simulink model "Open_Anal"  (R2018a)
settings: Solver=ode113  StartTime=0.0  StopTime=25000  FixedStep=0.1  RelTol=1e-3  EnableMultiTasking=on
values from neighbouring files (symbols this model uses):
  atto = [0, 0, -0]'*d2r    [run.m]
  ini = [wb0; atto; Hco]    [run.m]
  Kq1 = I22*ww^2 - 3*wo2*(I11-I33)    [run.m]
  Kq2 = 2*I22*zet*ww    [run.m]
  Kqi = 0.0005    [run.m]
  Kr1 = (0.1*I11*I33*zet^2/Hy0) - sqrt( ((0.01^zet^4*I11^2*I33^2)/Hy0^2)+(4*I11*I33*zet^2) )    [run.m]
  Kr2 = 0.05*Kr1    [run.m]
  Kr3 = 0.04*zet*(Kr2-Hy0) * sqrt(abs(Hy0/(I11*I33)))    [run.m]
  Tbs = (wo2)*[-2*I32, 3*I31, -I12]'    [run.m]
  Ts = 0.001    [run.m]    (also in runf.m = 0.0005)
  wb0 = [0.0, -wo, 0.0]'    [run.m]
undefined symbols (not defined in the file or in its folder): Avf, Bvf, Cvf, den, DiscIntNeverNeededParam, Dvf, num, Spacecraft, Wheel_Dynamics
libraries: simulink x3

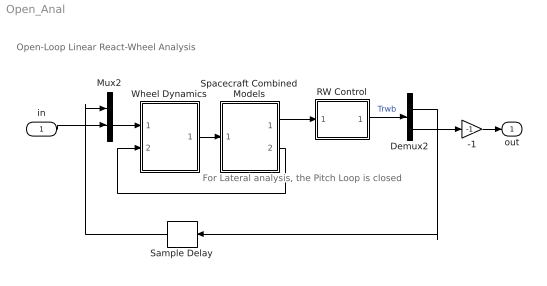
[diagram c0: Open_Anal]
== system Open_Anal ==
  note: Open-Loop Linear React-Wheel Analysis
  note: For Lateral analysis, the Pitch Loop is closed
  in : Inport
  -1 : Gain  Gain=-1
  Demux2 : Demux  Outputs=2
  Mux2 : Mux  Inputs=2
  RW Control : Subsystem
  Sample Delay : Delay  DelayLength=1  InputProcessing=Inherited  SampleTime=Ts
  Spacecraft Combined Models : Subsystem
  Wheel Dynamics : Subsystem
  out : Outport
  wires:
  -1/1 -> out/1
  Spacecraft Combined Models/2(wb) -> Wheel Dynamics/2(wb)
  Mux2/1 -> Wheel Dynamics/1(Twi)
  RW Control/1(Tc) -> Demux2/1  "Trwb"
  Spacecraft Combined Models/1(attit) -> RW Control/1(atti)
  Wheel Dynamics/1(Tcb) -> Spacecraft Combined Models/1(Trw)
  in/1 -> Mux2/2
  Demux2/2 -> -1/1
  Demux2/1 -> Sample Delay/1
  Sample Delay/1 -> Mux2/1

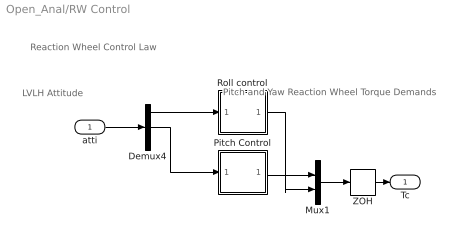
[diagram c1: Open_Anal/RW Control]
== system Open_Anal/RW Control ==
  note: Pitch and Yaw Reaction Wheel Torque Demands
  note: LVLH Attitude
  note: Reaction Wheel Control Law
  atti : Inport
  Demux4 : Demux  Outputs=3
  Mux1 : Mux  Inputs=2
  Pitch Control : Subsystem
  Roll control : Subsystem
  ZOH : ZeroOrderHold  SampleTime=Ts
  Tc : Outport
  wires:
  Demux4/1 -> Roll control/1(phi)
  Pitch Control/1(Tcy) -> Mux1/1
  Demux4/2 -> Pitch Control/1(the)
  Mux1/1 -> ZOH/1
  Roll control/1(Tcz) -> Mux1/2
  atti/1 -> Demux4/1
  ZOH/1 -> Tc/1

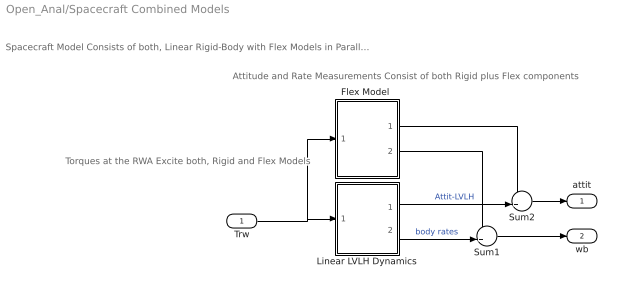
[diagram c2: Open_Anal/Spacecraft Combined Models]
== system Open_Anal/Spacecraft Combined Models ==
  note: Attitude and Rate Measurements Consist of both Rigid plus Flex components
  note: Spacecraft Model Consists of both, Linear Rigid-Body with Flex Models in Parallel
  note: Torques at the RWA Excite both, Rigid and Flex Models
  Trw : Inport
  "Flex Model " : Subsystem
  Linear LVLH Dynamics : Subsystem
  Sum1 : Sum  Inputs=++|
  Sum2 : Sum  Inputs=++|
  attit : Outport
  wb : Outport  Port=2
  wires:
  Trw/1 -> "Flex Model "/1(Trwi), Linear LVLH Dynamics/1(Tsc)
  "Flex Model "/1(att-flx) -> Sum2/1
  Linear LVLH Dynamics/1(atti-lv) -> Sum2/2  "Attit-LVLH"
  Sum2/1 -> attit/1
  Sum1/1 -> wb/1
  Linear LVLH Dynamics/2(wb) -> Sum1/2  "body rates"
  "Flex Model "/2(wb-flx) -> Sum1/1

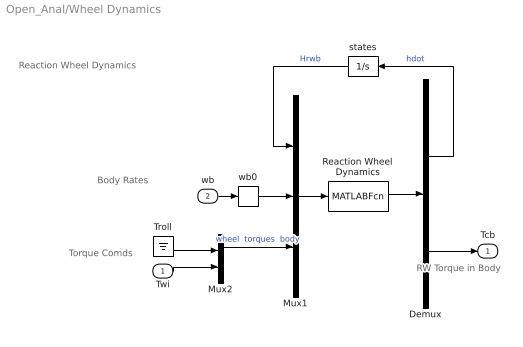
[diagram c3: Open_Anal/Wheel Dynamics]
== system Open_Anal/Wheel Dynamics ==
  note: Reaction Wheel Dynamics
  note: Body Rates
  note: RW Torque in Body
  note: Torque Comds
  Twi : Inport
  wb : Inport  Port=2
  Demux : Demux  Outputs=[3, 3]
  Mux1 : Mux  Inputs=[3, 3, 3]
  Mux2 : Mux  Inputs=[1,2]
  Reaction Wheel Dynamics : MATLABFcn  MATLABFcn=Wheel_Dynamics( u(1:3), u(4:6), u(7:9) )  OutputDimensions=3+3
  Troll : Ground
  states : Integrator
  wb0 : Memory  InitialCondition=wb0
  Tcb : Outport
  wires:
  states/1 -> Mux1/1  "Hrwb"
  Demux/1 -> states/1  "hdot"
  wb/1 -> wb0/1
  Mux2/1 -> Mux1/3  "wheel  torques  body"
  Demux/2 -> Tcb/1
  Reaction Wheel Dynamics/1 -> Demux/1
  Mux1/1 -> Reaction Wheel Dynamics/1
  Twi/1 -> Mux2/2
  Troll/1 -> Mux2/1
  wb0/1 -> Mux1/2

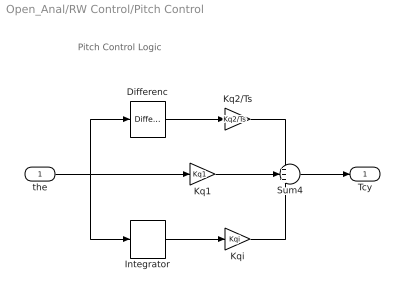
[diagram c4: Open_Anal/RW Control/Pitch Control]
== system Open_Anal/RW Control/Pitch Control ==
  note: Pitch Control Logic
  the : Inport
  Differenc : simulink/Discrete/Difference  ICPrevInput=0.0  OutDataType=sfix(16)  OutScaling=2^-10  DoSatur=off
  Integrator : DiscreteIntegrator  InitialCondition=atto(2)  SampleTime=Ts  ICPrevOutput=DiscIntNeverNeededParam  ICPrevScaledInput=DiscIntNeverNeededParam
  Kq1 : Gain  Gain=Kq1
  Kq2/Ts : Gain  Gain=Kq2/Ts
  Kqi : Gain  Gain=Kqi
  Sum4 : Sum  Inputs=+++
  Tcy : Outport
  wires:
  Kq1/1 -> Sum4/2
  Sum4/1 -> Tcy/1
  Kq2/Ts/1 -> Sum4/1
  the/1 -> Kq1/1, Integrator/1, Differenc/1
  Kqi/1 -> Sum4/3
  Integrator/1 -> Kqi/1
  Differenc/1 -> Kq2/Ts/1

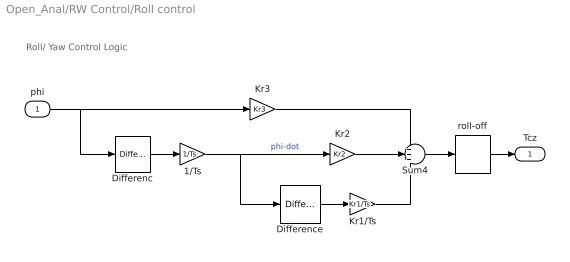
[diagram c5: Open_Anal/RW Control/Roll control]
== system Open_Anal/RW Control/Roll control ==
  note: Roll/ Yaw Control Logic
  phi : Inport
  1/Ts : Gain  Gain=1/Ts
  Differenc : simulink/Discrete/Difference  ICPrevInput=atto(1)  InputProcessing=Inherited  OutMin=[]  OutMax=[]  OutDataType=sfix(16)  OutScaling=2^-10  DoSatur=off
  Difference : simulink/Discrete/Difference  ICPrevInput=0.0  InputProcessing=Inherited  OutMin=[]  OutMax=[]  OutDataType=sfix(16)  OutScaling=2^-10  DoSatur=off
  Kr1/Ts : Gain  Gain=Kr1/Ts
  Kr2 : Gain  Gain=Kr2
  Kr3 : Gain  Gain=Kr3
  Sum4 : Sum  Inputs=+++
  roll-off : DiscreteTransferFcn  Numerator=[num]  Denominator=[den]  SampleTime=Ts
  Tcz : Outport
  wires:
  Kr3/1 -> Sum4/1
  Kr2/1 -> Sum4/2
  Kr1/Ts/1 -> Sum4/3
  phi/1 -> Kr3/1, Differenc/1
  Sum4/1 -> roll-off/1
  Difference/1 -> Kr1/Ts/1
  Differenc/1 -> 1/Ts/1
  1/Ts/1 -> Kr2/1, Difference/1  "phi-dot"
  roll-off/1 -> Tcz/1

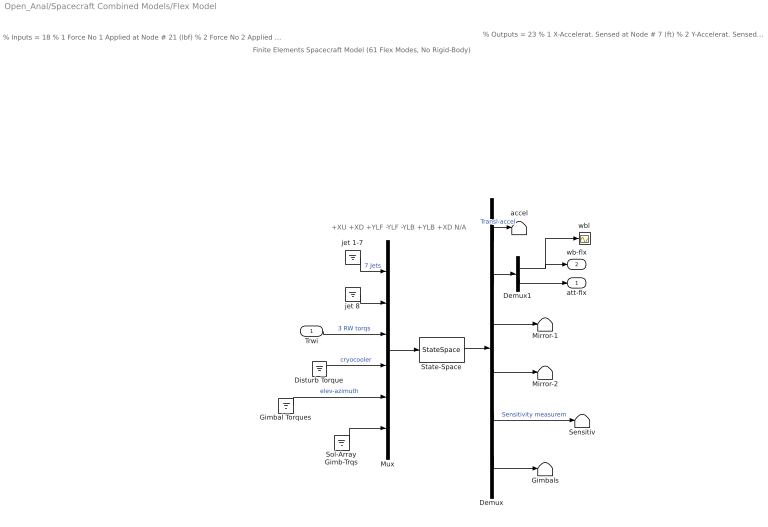
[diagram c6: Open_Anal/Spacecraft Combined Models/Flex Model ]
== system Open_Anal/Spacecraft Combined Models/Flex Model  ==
  note: Finite Elements Spacecraft Model (61 Flex Modes, No Rigid-Body)
  note: % Inputs = 18 % 1 Force No 1 Applied at Node # 21 (lbf) % 2 Force No 2 Applied at Node # 22 (lbf) % 3 Force No 3 Applied at Node # 23 (lbf) % 4 Force No 4 Applied at Node # 24 (lbf) % 5 Force No 5 Applied at Node # 25 (lbf) % 6 Force No 6 Applied at Node # 26 (lbf) % 7 Force No 7 Applied at Node # 27 (lbf) % 8 Force No 8 Applied at Node # 28 (lbf) % 9 Torque No 1 Applied at Node # 17 (ft-lb) % 10 Torque No 2 Applied at Node # 18 (ft-lb) % 11 Torque No 3 Applied at Node # 19 (ft-lb) % 12 Torque No 4 Applied at Node # 8 (ft-lb) % 13 Torque No 5 Applied at Node # 8 (ft-lb) % 14 Torque No 6 Applied at Node # 8 (ft-lb) % 15 Control Torque at Gimbal No 1 in (ft-lb) % 16 Control Torque at Gimbal No 2 in (ft-lb) % 17 Control Torque at Gimbal No 3 in (ft-lb) % 18 Control Torque at Gimbal No 4 in (ft-lb)
  note: % Outputs = 23 % 1 X-Accelerat. Sensed at Node # 7 (ft) % 2 Y-Accelerat. Sensed at Node # 7 (ft) % 3 X-Rot. Rate Sensed at Node # 6 (radian) % 4 Y-Rot. Rate Sensed at Node # 6 (radian) % 5 Z-Rot. Rate Sensed at Node # 6 (radian) % 6 X-Rotation Sensed at Node # 6 (radian) % 7 Y-Rotation Sensed at Node # 6 (radian) % 8 Z-Rotation Sensed at Node # 6 (radian) % 9 Y-Rotation Sensed at Node # 9 (radian) % 10 Z-Rotation Sensed at Node # 9 (radian) % 11 Y-Rotation Sensed at Node # 10 (radian) % 12 Z-Rotation Sensed at Node # 10 (radian) % 13 X-Rotation Sensed at Node # 11 (radian) % 14 Y-Rotation Sensed at Node # 12 (radian) % 15 Z-Rotation Sensed at Node # 13 (radian) % 16 Rotation Angle at Gimbal No 1 in (radians) % 17 Rotation Rate at Gimbal No 1 in (rad/sec) % 18 Rotation Angle at Gimbal No 2 in (radians) % 19 Rotation Rate at Gimbal No 2 in (rad/sec) % 20 Rotation Angle at Gimbal No 3 in (radians) % 21 Rotation Rate at Gimbal No 3 in (rad/sec) % 22 Rotation Angle at Gimbal No 4 in (radians) % 23 Rotation Rate at Gimbal No 4 in (rad/sec)
  note: +XU +XD +YLF -YLF -YLB +YLB +XD N/A
  Trwi : Inport
  Demux : Demux  Outputs="[2, 6, 2,2,3,  8]"
  Demux1 : Demux  Outputs=[3, 3]
  Disturb Torque : Ground
  Gimbal Torques : Ground
  Gimbals : Terminator
  Mirror-1 : Terminator
  Mirror-2 : Terminator
  Mux : Mux  Inputs=[7,1,3,3,2,2]
  Sensitiv : Terminator
  Sol-Array Gimb-Trqs : Ground
  State-Space : StateSpace  A=Avf  B=Bvf  C=Cvf  D=Dvf  InitialCondition=0
  accel : Terminator
  jet 1-7 : Ground
  jet 8 : Ground
  wbl : Scope
  att-flx : Outport
  wb-flx : Outport  Port=2
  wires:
  Demux/6 -> Gimbals/1
  Gimbal Torques/1 -> Mux/5  "elev-azimuth"
  Demux/1 -> accel/1  "Transl-accel"
  State-Space/1 -> Demux/1
  Demux/2 -> Demux1/1
  Demux1/1 -> wbl/1, wb-flx/1
  Mux/1 -> State-Space/1
  jet 1-7/1 -> Mux/1  "7 Jets"
  jet 8/1 -> Mux/2
  Trwi/1 -> Mux/3  "3 RW torqs"
  Disturb Torque/1 -> Mux/4  "cryocooler"
  Sol-Array Gimb-Trqs/1 -> Mux/6
  Demux/5 -> Sensitiv/1  "Sensitivity measurem"
  Demux/3 -> Mirror-1/1
  Demux/4 -> Mirror-2/1
  Demux1/2 -> att-flx/1

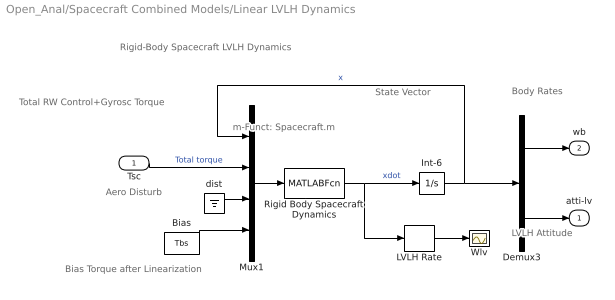
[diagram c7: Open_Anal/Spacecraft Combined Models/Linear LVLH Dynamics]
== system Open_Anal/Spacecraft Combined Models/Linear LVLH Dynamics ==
  note: State Vector
  note: Rigid-Body Spacecraft LVLH Dynamics
  note: Total RW Control+Gyrosc Torque
  note: Aero Disturb
  note: Bias Torque after Linearization
  note: Body Rates
  note: LVLH Attitude
  note: m-Funct: Spacecraft.m
  Tsc : Inport
  Bias : Constant  Value=Tbs
  Demux3 : Demux  Outputs=[3, 3]
  Int-6 : Integrator  InitialCondition=ini
  LVLH Rate : Selector  InputPortWidth=6  IndexOptions=Index vector (dialog)  Indices=[4:6]  OutputSizes=1
  Mux1 : Mux  Inputs=[6, 3, 3, 3]
  Rigid Body Spacecraft Dynamics : MATLABFcn  MATLABFcn=Spacecraft( u(1:6), u(7:9) , u(10:12), u(13:15) )  OutputDimensions=6
  Wlv : Scope
  dist : Ground
  atti-lv : Outport
  wb : Outport  Port=2
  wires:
  Mux1/1 -> Rigid Body Spacecraft Dynamics/1
  Demux3/2 -> atti-lv/1
  Demux3/1 -> wb/1
  Int-6/1 -> Demux3/1, Mux1/1  "x"
  Tsc/1 -> Mux1/2  "Total torque"
  Rigid Body Spacecraft Dynamics/1 -> Int-6/1, LVLH Rate/1  "xdot"
  LVLH Rate/1 -> Wlv/1
  Bias/1 -> Mux1/4
  dist/1 -> Mux1/3
